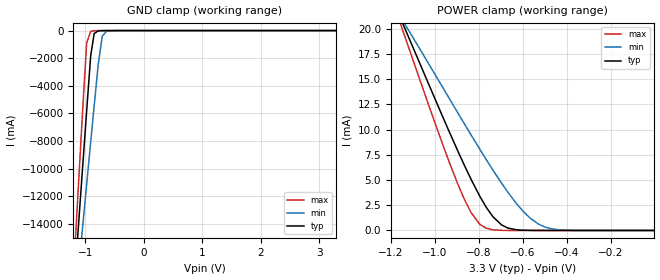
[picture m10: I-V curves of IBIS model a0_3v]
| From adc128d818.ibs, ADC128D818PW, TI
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[Model] a0_3v
Model_type Input
Vinh = 2.0V
Vinl = 0.8V
C_comp   2.30pF   2.02pF   2.64pF
[Voltage Range]   3.3V   3.0V   3.6V
[Temperature Range]   25.0   125.0   -40.0
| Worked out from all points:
|   GND clamp passes 1 mA (typ) near -0.64 V on its own axis
|   POWER clamp passes 1 mA (typ) near -0.72 V on its own axis
[GND Clamp]
-3.3V     -143.8A    -115.1A    -176.2A
-1.171V   -17.65A    -20.12A    -15.61A
-1.102V   -13.47A    -16.96A    -10.33A
-1.043V   -9.928A    -14.27A    -5.851A
-973.5mV  -5.843A    -11.15A    -904.3mA
-904.2mV  -1.818A    -8.067A    -51.13mA
-844.8mV  -212.8mA   -5.459A    -10.53mA
-775.5mV  -24.49mA   -2.452A    -2.604mA
-706.2mV  -4.459mA   -401.4mA   -511.5uA
-636.9mV  -871.5uA   -63.32mA   -72.55uA
-438.9mV  -3.537uA   -616.8uA   -60.87nA
3.293V    693.7pA    0A         688pA
[POWER Clamp]
-3.3V     87.45mA    70.01mA    101.4mA
-1.162V   21.29mA    21.35mA    20.8mA
-1.132V   19.79mA    20.28mA    18.93mA
-1.102V   18.28mA    19.21mA    17.06mA
-894.3mV  7.82mA     11.62mA    4.533mA
-834.9mV  5.06mA     9.467mA    1.764mA
-795.3mV  3.388mA    8.054mA    610.1uA
-696.3mV  550uA      4.691mA    13.26uA
-597.3mV  24.18uA    1.881mA    403.9nA
-528mV    2.48uA     631.2uA    36.5nA
-429mV    102.3nA    62.71uA    1.71nA
-3.3mV    696.2pA    7.015nA    764.2pA
